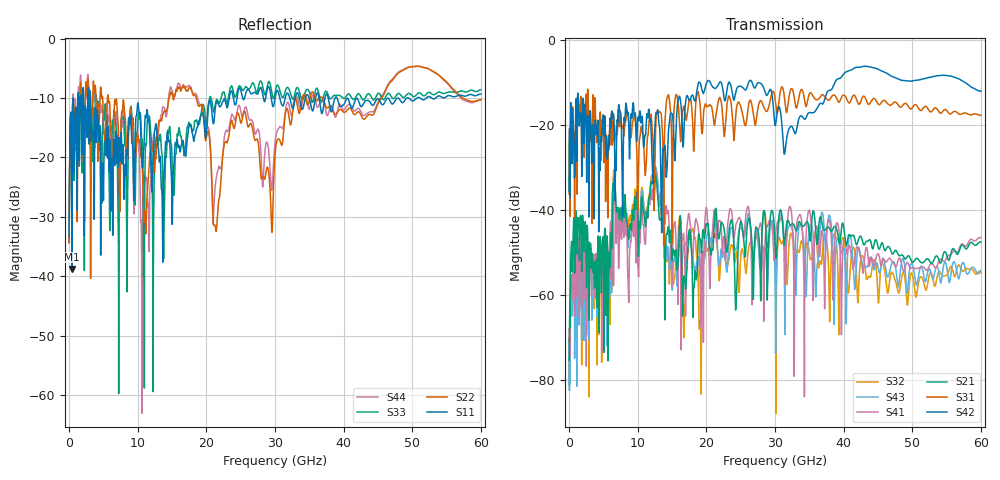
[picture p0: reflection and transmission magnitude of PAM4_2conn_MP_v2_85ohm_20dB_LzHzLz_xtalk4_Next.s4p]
! Info: Touchstone file created by Circ.  Input file=FAB50GbE_2conn_Midplane_Examax_Topo2_v2_85ohm_20dB_LzHzLz.circ
# Hz S RI R 50
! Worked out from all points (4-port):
!   6000 points, 10 MHz to 60 GHz, reference 50 ohm
!   strongest paths, dB at 10 MHz, 15.01 GHz, 30.01 GHz, 45.01 GHz, 60 GHz:
!     S42: -35.6, -17.4, -20.2, -7.0, -12.1
!     S31: -36.3, -34.2, -13.8, -15.1, -17.8
!     S21: -75.4, -51.8, -47.4, -48.7, -47.6
!     S41: -68.0, -57.1, -48.8, -50.4, -46.6
!     S43: -71.0, -57.2, -55.6, -53.5, -54.3
!     S32: -74.7, -56.5, -52.5, -60.5, -54.9
!   lowest |S11| = -38.8 dB at 410 MHz (marker M1), VSWR 1.02, Z = 51 - j0.542 ohm
!   |S11| at or under -10 dB: start of sweep to 1.29 GHz; 3.125 GHz to 23.34 GHz (20.22 GHz wide, 153 % of centre); 39.04 GHz to 49.25 GHz (10.21 GHz wide, 23.1 % of centre)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
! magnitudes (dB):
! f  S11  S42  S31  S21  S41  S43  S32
! 10 MHz  -33.2  -35.6  -36.3  -75.4  -68.0  -71.0  -74.7
! 410 MHz  -38.8  -28.5  -29.1  -48.1  -58.5  -63.4  -56.8
! 12.69 GHz  -14.4  -17.2  -18.5  -33.0  -32.3  -30.4  -30.7
! 19.11 GHz  -13.2  -10.2  -15.6  -46.9  -56.1  -55.6  -66.2
! 21.27 GHz  -12.0  -11.5  -19.4  -40.9  -40.7  -42.3  -45.8
! 28.45 GHz  -10.6  -11.8  -16.2  -40.4  -53.4  -48.7  -40.2
! 60 GHz  -9.4  -12.1  -17.8  -47.6  -46.6  -54.3  -54.9
